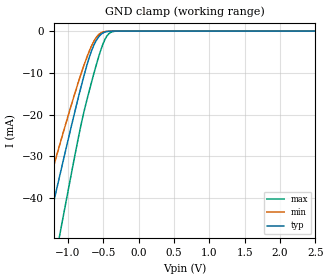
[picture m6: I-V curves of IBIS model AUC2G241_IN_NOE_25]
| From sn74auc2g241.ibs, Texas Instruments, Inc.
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[Model]   AUC2G241_IN_NOE_25
Model_type  Input
Vinl=0.7
Vinh=1.7
| variable   typ   min   max
C_comp   2.55pF   1.99pF   2.92pF
[Temperature Range]   40   100   -40
| Ambient temperature   25   85   -40
[Voltage range]   2.5   2.3   2.7
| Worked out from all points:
|   GND clamp passes 1 mA (typ) near -0.55 V on its own axis
[GND Clamp]
| AUC2G241_IN_NOE_25
|   Voltage   I(typ)   I(min)   I(max)
-3.6V     -223.1mA   -186.8mA   -268.3mA
-1.485V   -62.1mA    -49.68mA   -81.81mA
-1.435V   -58.34mA   -46.58mA   -77.34mA
-1.3V     -48.22mA   -38.26mA   -65.26mA
-1.115V   -34.53mA   -27.12mA   -48.68mA
-830mV    -14.34mA   -11.03mA   -23.64mA
-720mV    -7.475mA   -5.71mA    -15.68mA
-625mV    -3.066mA   -2.194mA   -9.633mA
-525mV    -682.6uA   -365uA     -4.021mA
-430mV    -73.19uA   -35.15uA   -776.9uA
-325mV    -3.339uA   -2.023uA   -30.74uA
2.5V      328.6pA    416.1pA    485.4pA
